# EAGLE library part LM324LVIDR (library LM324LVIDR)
4-Channel Industry Standard Low Voltage Operational Amplifier Source: Datasheet
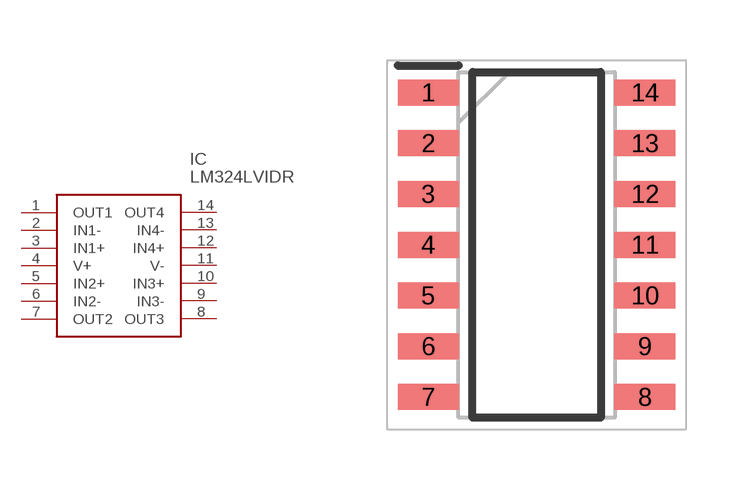
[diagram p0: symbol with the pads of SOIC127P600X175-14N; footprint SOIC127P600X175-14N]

Designator prefix IC

## LM324LVIDR (Arrow_Part_Number: LM324LVIDR; Arrow_Price-Stock: https://www.arrow.com/en/products/lm324lvidr/texas-instruments; Description: 4-Channel Industry Standard Low Voltage Operational Amplifier; Height: 1.75mm; Manufacturer_Name: Texas Instruments; Manufacturer_Part_Number: LM324LVIDR; Mouser_Part_Number: 595-LM324LVIDR; Mouser_Price-Stock: https://www.mouser.co.uk/ProductDetail/Texas-Instruments/LM324LVIDR/?qs=qSfuJ%252Bfl%2Fd62Uwb7PBNJ4g%3D%3D)  [SOIC127P600X175-14N]
1  OUT1
2  IN1-
3  IN1+
4  V+
5  IN2+
6  IN2-
7  OUT2
8  OUT3
9  IN3-
10  IN3+
11  V-
12  IN4+
13  IN4-
14  OUT4

## Footprint SOIC127P600X175-14N (pad centres in mm)
LM324LVIDR-1
smd 1.525 x 0.65: 1 -2.712,3.81; 2 -2.712,2.54; 3 -2.712,1.27; 4 -2.712,0; 5 -2.712,-1.27; 6 -2.712,-2.54; 7 -2.712,-3.81; 8 2.712,-3.81; 9 2.712,-2.54; 10 2.712,-1.27; 11 2.712,0; 12 2.712,1.27; 13 2.712,2.54; 14 2.712,3.81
